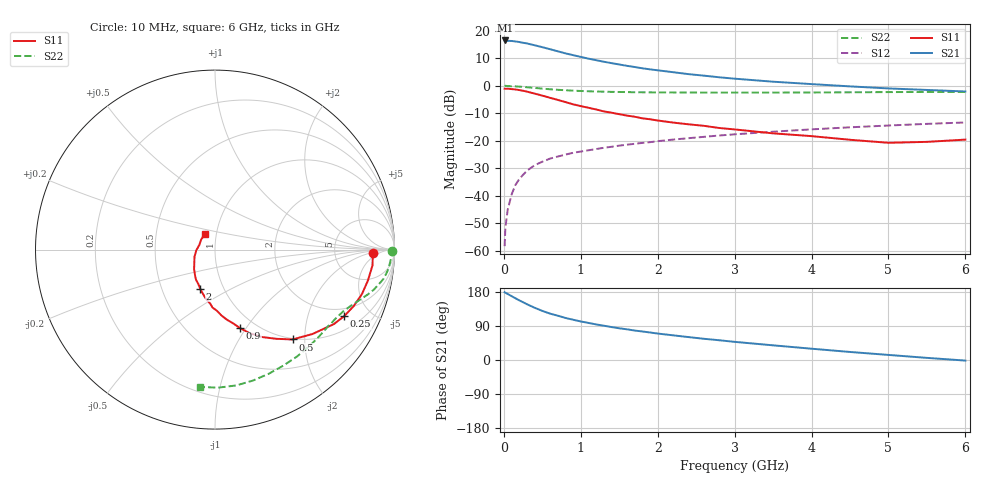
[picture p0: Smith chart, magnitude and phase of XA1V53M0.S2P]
! SIEMENS Discrete & RF Semiconductors
! BFY180
! Si NPN RF Bipolar Junction Transistor in MICRO-X
! VCE = 1.5 V  IC = 3 mA
! Common Emitter S-Parameters:  May  1997
# GHz  S  MA  R  50
!  f  S11  S21  S12  S22
! GHz  MAG  ANG  MAG  ANG  MAG  ANG  MAG  ANG
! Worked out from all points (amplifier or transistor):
!   36 points, 10 MHz to 6 GHz, reference 50 ohm
!   highest |S21| = 16.5 dB at 20 MHz (marker M1)
!   |S21| within 3 dB of that: start of sweep to 575.3 MHz
!   unconditionally stable (mu >= 1): 1.277 GHz to end of sweep
!   at 250 MHz: K = 0.26, MSG = 24.0 dB, |S12| = -32.4 dB
!   at 1.4 GHz: K = 1.04, MAG = 13.9 dB, |S12| = -22.2 dB
!   at 6 GHz: K = 1.20, MAG = 2.9 dB, |S12| = -13.4 dB
!   S11 on the Smith chart (normalised r, x): 10 MHz: 16, -3; 250 MHz: 1.59, -3.43; 500 MHz: 0.98, -1.75; 900 MHz: 0.85, -0.94; 2 GHz: 0.78, -0.36; 6 GHz: 0.88, +0.16
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0.01  0.8825 -1.2  6.581 178.9  0.0012 86.5  0.9858 -0.3
0.02  0.8796 -2.1  6.671 177.6  0.0026 96.7  0.9972 -0.9
0.05  0.8819 -5.7  6.561 174.3  0.0055 85.2  0.9854 -2.1
0.1  0.8694 -11.4  6.532 168.6  0.0104 83.1  0.9777 -4.2
0.2  0.8343 -22.2  6.248 157.4  0.0199 77.8  0.9628 -8.1
0.25  0.8095 -27.3  6.052 152.4  0.0239 74.8  0.9527 -9.8
0.3  0.7814 -32.1  5.886 147.2  0.0283 71.4  0.9381 -11.4
0.4  0.7183 -40.9  5.456 137.9  0.0357 67.0  0.913 -14.1
0.5  0.6614 -49.2  5.034 129.6  0.0414 62.8  0.8856 -16.5
0.6  0.6031 -55.5  4.625 122.4  0.0471 60.5  0.8621 -18.4
0.7  0.5527 -61.8  4.241 117.0  0.0514 57.9  0.8438 -20.1
0.8  0.5045 -67.4  3.884 111.0  0.0557 56.2  0.8274 -21.6
0.9  0.4594 -72.3  3.605 106.3  0.0601 54.6  0.8135 -23.1
1.1  0.3972 -80.2  3.113 97.8  0.0668 53.0  0.7922 -25.8
1.5  0.3033 -94.9  2.437 83.7  0.0812 50.5  0.7694 -31.4
2  0.2328 -110.7  1.909 69.8  0.0979 48.0  0.7562 -38.4
2.2  0.2135 -115.8  1.763 65.1  0.1046 46.6  0.7544 -41.4
2.8  0.1701 -131.9  1.425 52.1  0.1241 43.1  0.7505 -49.8
3.5  0.1359 -148.1  1.184 38.7  0.1456 38.2  0.7503 -59.6
4.5  0.1038 -178.4  0.973 21.2  0.175 30.6  0.7596 -73.8
5.5  0.0951 144.2  0.838 5.6  0.2021 22.5  0.7694 -88.7
6  0.1045 123.2  0.786 -1.5  0.2145 18.1  0.7697 -96.2
